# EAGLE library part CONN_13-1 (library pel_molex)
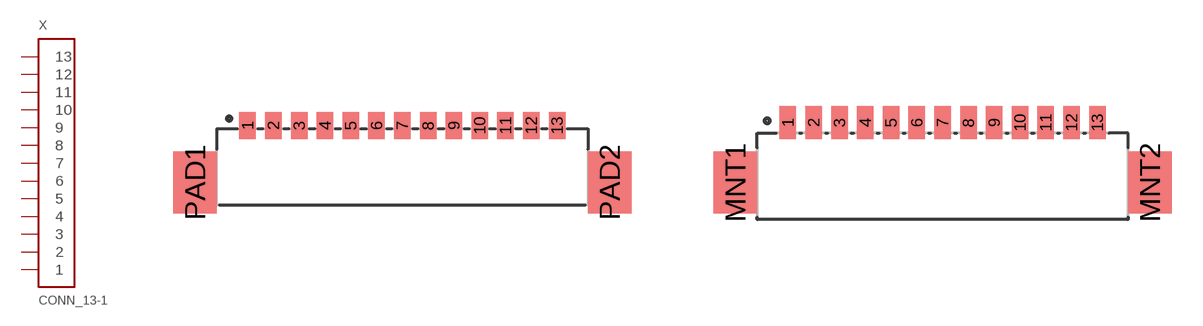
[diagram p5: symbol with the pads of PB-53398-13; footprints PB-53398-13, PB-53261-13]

Designator prefix X

## CONN_13-1-53398  [PB-53398-13]
1  1
2  2
3  3
4  4
5  5
6  6
7  7
8  8
9  9
10  10
11  11
12  12
13  13

## CONN_13-1-53261  [PB-53261-13]
Pads as for PB-53398-13

## CONN_13-1-53047  [PB-53047-13]
Pads as for PB-53398-13

## Footprint PB-53398-13 (pad centres in mm)
smd 0.8 x 1.3: 1 -7.5,1.25; 2 -6.25,1.25; 3 -5,1.25; 4 -3.75,1.25; 5 -2.5,1.25; 6 -1.25,1.25; 7 0,1.25; 8 1.25,1.25; 9 2.5,1.25; 10 3.75,1.25; 11 5,1.25; 12 6.25,1.25; 13 7.5,1.25
smd 2.1 x 3: PAD1 -10.05,-1.5; PAD2 10.05,-1.5

## Footprint PB-53261-13 (pad centres in mm)
smd 0.8 x 1.6: 1 -7.5,1.1; 2 -6.25,1.1; 3 -5,1.1; 4 -3.75,1.1; 5 -2.5,1.1; 6 -1.25,1.1; 7 0,1.1; 8 1.25,1.1; 9 2.5,1.1; 10 3.75,1.1; 11 5,1.1; 12 6.25,1.1; 13 7.5,1.1
smd 2.1 x 3: MNT1 -10.05,-1.8; MNT2 10.05,-1.8

## Footprint PB-53047-13 (pad centres in mm)
drill 0.5: 1 -7.5,0; 2 -6.25,0; 3 -5,0; 4 -3.75,0; 5 -2.5,0; 6 -1.25,0; 7 0,0; 8 1.25,0; 9 2.5,0; 10 3.75,0; 11 5,0; 12 6.25,0; 13 7.5,0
